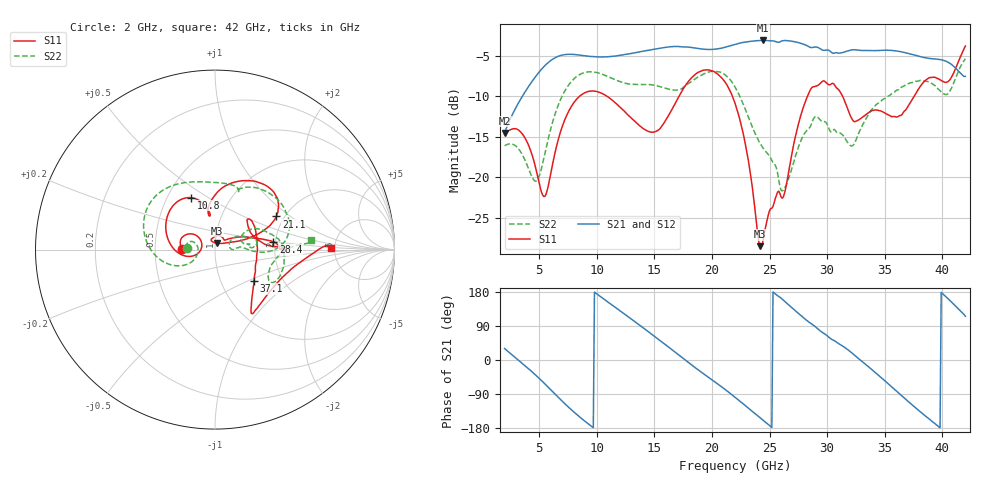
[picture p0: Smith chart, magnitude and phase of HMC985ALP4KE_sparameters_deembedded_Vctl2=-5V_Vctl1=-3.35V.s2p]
!s2p File: Measurements: S11, S21, S12, S22
# GHz S dB R 50.0
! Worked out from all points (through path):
!   401 points, 2 GHz to 42 GHz, reference 50 ohm
!   highest |S21| = -3.14 dB at 24.4 GHz (marker M1); lowest = -14.5 dB at 2 GHz (marker M2)
!   lowest |S11| = -28.5 dB at 24.2 GHz (marker M3), VSWR 1.08, Z = 50.8 + j3.7 ohm
!   |S11| at or under -10 dB: start of sweep to 8.533 GHz; 10.85 GHz to 17.16 GHz (6.301 GHz wide, 45 % of centre); 21.76 GHz to 28.3 GHz (6.535 GHz wide, 26.1 % of centre)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
!   |S22| runs from -21.7 to -5.4 dB; largest |S21 - S12| = 0.00068
!   S11 on the Smith chart (normalised r, x): 2 GHz: 0.69, +0.01; 10.8 GHz: 0.66, +0.42; 21.1 GHz: 1.82, +0.79; 28.4 GHz: 1.95, +0.19; 37.1 GHz: 1.43, -0.54; 42 GHz: 4.61, +0.10
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2  -14.74 178.6  -14.55 30.2  -14.55 30.2  -16.14 176.8
4.7  -18.90 143.2  -7.58 -39.9  -7.58 -39.9  -20.53 -179.2
5.5  -22.38 173.8  -6.24 -63.1  -6.25 -63.1  -17.09 -152.9
6.9  -14.21 -172.4  -4.98 -105.6  -4.99 -105.6  -10.29 -168.8
8.7  -9.82 145.5  -4.98 -155.0  -4.99 -155.0  -7.22 154.0
10.8  -9.95 114.5  -5.17 156.7  -5.17 156.7  -7.50 120.5
13.3  -13.12 99.4  -4.66 101.4  -4.66 101.4  -8.56 86.6
15.4  -14.15 100.5  -4.13 53.5  -4.13 53.5  -8.80 69.3
18  -8.12 73.5  -3.97 -7.6  -3.97 -7.6  -8.42 65.4
21.1  -8.21 28.4  -4.00 -76.7  -4.00 -76.7  -7.35 15.7
22  -10.88 21.1  -3.62 -98.2  -3.63 -98.2  -8.88 2.5
24.2  -28.54 76.3  -3.15 -152.8  -3.15 -152.7  -15.89 3.4
24.4  -28.08 97.6  -3.14 -157.8  -3.14 -157.8  -16.35 4.8
26.2  -22.45 44.2  -3.16 157.9  -3.16 157.9  -21.61 18.0
28.4  -9.67 7.6  -3.90 100.5  -3.90 100.5  -14.02 18.8
28.7  -8.92 2.7  -4.02 94.4  -4.02 94.4  -13.19 17.5
30.6  -8.55 0.8  -4.71 51.5  -4.71 51.5  -14.12 8.9
32.4  -13.17 26.6  -4.29 12.0  -4.29 12.0  -15.75 26.0
35.4  -12.38 13.4  -4.36 -65.5  -4.36 -65.4  -9.95 16.3
37.1  -11.08 -38.8  -4.77 -111.2  -4.77 -111.1  -8.46 2.1
39.7  -7.91 -54.3  -5.48 -176.5  -5.48 -176.5  -9.21 -29.9
42  -3.83 0.6  -7.58 115.3  -7.58 115.3  -5.39 5.9
